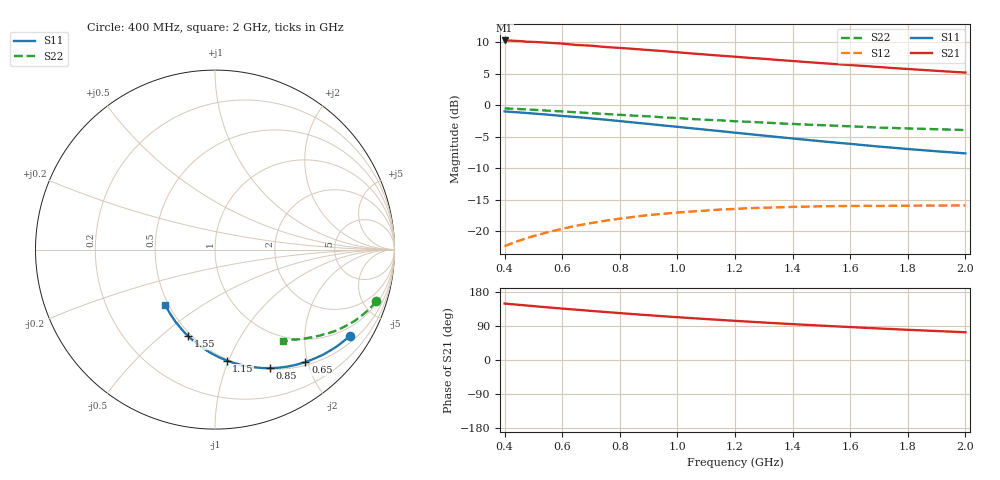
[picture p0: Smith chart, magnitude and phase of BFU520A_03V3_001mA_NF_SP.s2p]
! Filename:  P:\Prog\Test\Noise\ATS_data\Testdata_Net\06 Compressed Noise after Statistics\BFU520A_APG2013_30_A05_03p3V_001mA_NF_CM01_D.sf
! Date/Time: Wed 24/Apr/2013 20:06:15
! BFU520A_APG2013_30_A05_03p3V_1to20mA_NF_CM01_Bias1_R.sf
! Noise Parameter Data File
! BFU520A_APG2013_30_A05_03p3V_1to20mA_NF_CM01
! Date/time: Thu Apr 11 00:04:13 2013
! freq range =  0.4000 to  2.0000 GHz, 37 points
! bias range =  1.0000 to 19.9950 mA, 8 points
! bias supplies used: 1 1 0 0 0 0
! VAR bias_mode= 1  ! Specify V_out, I_out
! VAR bias_var = 1  ! Bias variable = I_out
! VAR V_out= 3.301000
! VAR I_out= 1.000000
! VAR V_in= 0.793800
! VAR I_in= 0.010800
! Device data file deembeded for feedlines and parallel
! Original file: \06 Compressed Noise after Statistics\BFU520A_APG2013_30_A05_03p3V_001mA_NF_CM01_R.sf
! Feed-files: PR017V01_150413_Feed1.s2p, PR017V01_150413_Feed2.s2p
! Parallel-file: PR017V01_150413_Par.s2p
# MHz S MA R 50
!  Freq-MHz  S11-mag  S11-arg  S21-mag  S21-arg  S12-mag  S12-arg  S22-mag  S22-arg
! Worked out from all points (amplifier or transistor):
!   37 points, 400 MHz to 2 GHz, reference 50 ohm
!   highest |S21| = 10.2 dB at 400 MHz (marker M1)
!   |S21| within 3 dB of that: start of sweep to 1.326 GHz
!   unconditionally stable (mu >= 1): nowhere
!   at 500 MHz: K = 0.23, MSG = 15.4 dB, |S12| = -20.7 dB
!   at 1.1 GHz: K = 0.49, MSG = 12.3 dB, |S12| = -16.7 dB
!   at 2 GHz: K = 0.87, MSG = 10.5 dB, |S12| = -15.9 dB
!   lowest NFmin = 0.54 dB at 420 MHz
!   S11 on the Smith chart (normalised r, x): 400 MHz: 0.70, -3.28; 650 MHz: 0.55, -1.96; 850 MHz: 0.51, -1.44; 1.15 GHz: 0.49, -0.98; 1.55 GHz: 0.48, -0.62; 2 GHz: 0.48, -0.36
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400  0.8909 -32.6  3.248 149.1  0.07649 69.1  0.9425 -17.7
440  0.878 -35.8  3.222 146.2  0.08292 67.2  0.9333 -19.2
460  0.8716 -37.4  3.204 144.9  0.08601 66.4  0.9288 -20.0
480  0.8652 -38.8  3.17 143.6  0.08893 65.5  0.9228 -20.8
500  0.8576 -40.4  3.164 142.2  0.09186 64.6  0.9181 -21.5
550  0.8401 -44.2  3.117 138.9  0.09863 62.5  0.9037 -23.3
600  0.8206 -47.9  3.068 135.7  0.105 60.6  0.8903 -25.0
650  0.8043 -51.2  2.99 132.7  0.1111 58.7  0.8775 -26.6
700  0.7848 -54.9  2.953 129.6  0.1165 57.0  0.8635 -28.1
750  0.7669 -58.2  2.881 126.7  0.1217 55.3  0.8507 -29.6
800  0.7474 -61.7  2.836 123.8  0.1263 53.8  0.8375 -31.0
850  0.7279 -65.1  2.782 120.9  0.1306 52.2  0.8249 -32.4
950  0.6902 -71.7  2.677 115.5  0.1379 49.5  0.7998 -34.9
1050  0.6557 -77.8  2.562 110.5  0.1438 47.2  0.7758 -37.2
1150  0.6217 -84.0  2.46 105.7  0.1492 45.1  0.7569 -39.2
1200  0.605 -87.0  2.415 103.4  0.1508 44.3  0.7453 -40.3
1350  0.5585 -95.7  2.276 96.7  0.1552 42.1  0.7173 -43.1
1500  0.5172 -104.3  2.149 90.7  0.1581 40.5  0.6936 -45.7
1550  0.505 -107.1  2.111 88.8  0.1589 40.1  0.6871 -46.6
1750  0.4597 -118.3  1.964 81.4  0.1598 39.6  0.6592 -49.7
1850  0.4402 -123.7  1.899 78.0  0.1603 39.5  0.6494 -51.3
2000  0.4149 -132.0  1.809 73.2  0.1606 40.4  0.6347 -53.5
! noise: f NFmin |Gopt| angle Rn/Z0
400  0.5572  0.6547  17.33  0.3564
460  0.5693  0.6594  21.31  0.3697
600  0.6058  0.6164  26.47  0.3643
800  0.6417  0.6111  38.48  0.278
1000  0.6859  0.6044  49.9  0.2624
1200  0.7582  0.5911  59.43  0.2692
1400  0.7588  0.5292  70.05  0.2378
1600  0.8268  0.5321  83.34  0.177
1800  0.6788  0.4724  95.08  0.1447
2000  0.8206  0.4461  105.8  0.1333
